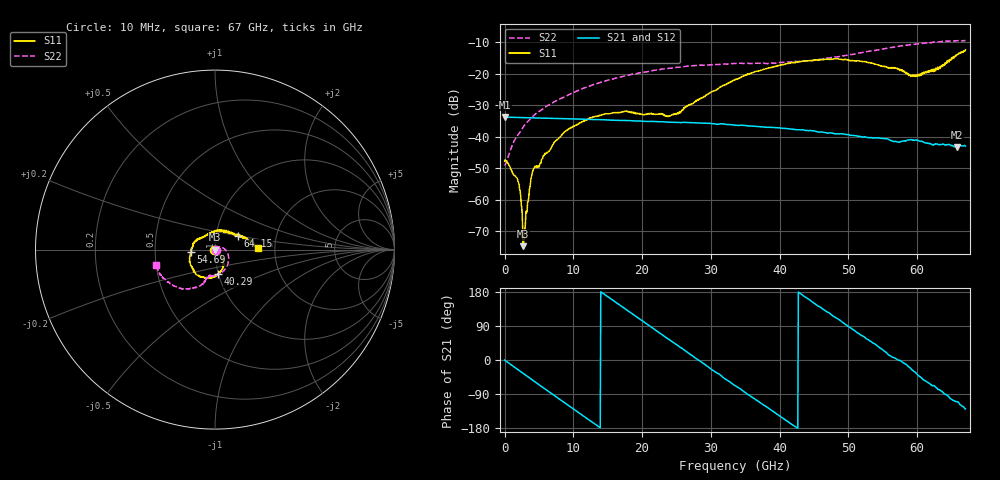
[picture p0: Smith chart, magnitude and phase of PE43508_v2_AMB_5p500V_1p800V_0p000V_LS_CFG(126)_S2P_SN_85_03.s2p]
!Keysight Technologies,N5227A,US51270237,A.10.43.00
!Date: Wednesday, August 22, 2018 17:19:52
!Correction: S11(Full 2 Port(1,3))
!S31(Full 2 Port(1,3))
!S13(Full 2 Port(1,3))
!S33(Full 2 Port(1,3))
!S2P File: Measurements: S11, S31, S13, S33:
# Hz S  dB  R 50
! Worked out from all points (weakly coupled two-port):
!   801 points, 10 MHz to 67 GHz, reference 50 ohm
!   highest |S21| = -33.74 dB at 10 MHz (marker M1); lowest = -43.2 dB at 65.74 GHz (marker M2)
!   lowest |S11| = -74.9 dB at 2.69 GHz (marker M3), VSWR 1.00, Z = 50 + j0.00317 ohm
!   |S11| at or under -10 dB: start of sweep to end of sweep
!   |S22| runs from -49.0 to -9.4 dB; largest |S21 - S12| = 0.00013
!   S11 on the Smith chart (normalised r, x): 10 MHz: 0.99, -0.00; 40.29 GHz: 0.99, -0.28; 54.69 GHz: 0.77, -0.02; 64.15 GHz: 1.27, +0.19; 67 GHz: 1.63, +0.03
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1e7  -47.77 -175.6  -33.74 -0.3  -33.74 -0.3  -48.91 -1.4
1.935962e9  -54.07 160.3  -33.87 -25.6  -33.87 -25.6  -39.51 47.4
2.187175e9  -56.72 166.8  -33.89 -28.9  -33.89 -28.9  -38.73 46.4
2.6896e9  -74.86 169.9  -33.92 -35.4  -33.92 -35.4  -36.98 44.3
3.02455e9  -68.08 36.2  -33.94 -39.8  -33.94 -39.8  -35.95 44.0
3.861925e9  -53.14 -33.9  -33.99 -50.5  -33.99 -50.5  -34.15 39.4
4.36435e9  -49.81 -21.1  -34.01 -56.9  -34.02 -57.0  -33.04 37.7
8.634962e9  -38.70 -59.3  -34.26 -111.6  -34.26 -111.6  -27.42 15.3
1.123082e10  -35.23 -67.7  -34.41 -144.7  -34.42 -144.7  -24.82 -0.9
1.74274e10  -31.98 -87.8  -34.82 136.4  -34.82 136.4  -20.68 -34.2
2.236791e10  -32.77 -82.6  -35.23 73.5  -35.23 73.4  -18.71 -57.1
2.513125e10  -32.39 -64.6  -35.46 38.9  -35.45 38.8  -17.86 -67.8
3.3505e10  -21.88 -55.8  -36.32 -67.7  -36.32 -67.7  -16.70 -93.3
4.028774e10  -17.16 -83.3  -37.28 -151.5  -37.28 -151.4  -16.37 -103.0
4.472582e10  -15.74 -106.8  -38.11 153.5  -38.10 153.5  -15.73 -105.4
4.841028e10  -15.18 -126.9  -39.11 109.1  -39.12 109.0  -14.59 -107.8
5.469059e10  -17.49 -174.8  -40.53 30.3  -40.50 30.1  -12.16 -119.4
5.586291e10  -18.17 171.5  -40.86 13.0  -40.87 13.1  -11.70 -122.8
5.979858e10  -20.34 113.3  -41.03 -33.9  -41.03 -34.2  -10.53 -135.2
6.415292e10  -16.67 30.2  -42.63 -90.6  -42.68 -90.6  -9.61 -152.6
6.574394e10  -14.11 13.6  -43.23 -110.3  -43.32 -110.7  -9.44 -159.1
6.7e10  -12.37 1.7  -42.99 -129.0  -43.08 -129.2  -9.35 -165.4
